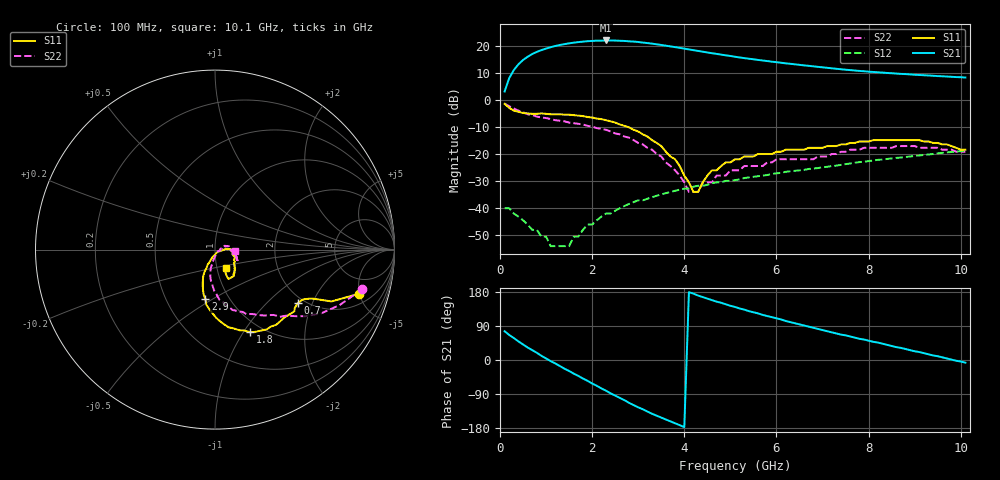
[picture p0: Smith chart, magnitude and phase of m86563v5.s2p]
!  MGA-86563 S PARAMETERS
!  Vd = 5 V  LAST UPDATED 12-19-94
# ghz s ma r 50
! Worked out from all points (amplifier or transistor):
!   101 points, 100 MHz to 10.1 GHz, reference 50 ohm
!   highest |S21| = 21.9 dB at 2.3 GHz (marker M1)
!   |S21| within 3 dB of that: 1 GHz to 3.993 GHz (2.992 GHz wide, 120 % of centre)
!   unconditionally stable (mu >= 1): start of sweep to end of sweep
!   at 1.7 GHz: K = 9.49, MAG = 23.1 dB, |S12| = -50.5 dB
!   at 5.1 GHz: K = 2.52, MAG = 15.9 dB, |S12| = -29.6 dB
!   at 10.1 GHz: K = 1.78, MAG = 8.3 dB, |S12| = -18.7 dB
!   lowest NFmin = 1.52 dB at 1.5 GHz
!   S11 on the Smith chart (normalised r, x): 100 MHz: 2.97, -4.96; 700 MHz: 1.84, -1.58; 1.8 GHz: 0.87, -1.07; 2.9 GHz: 0.78, -0.46; 10.1 GHz: 1.11, -0.23
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0.1  0.84 -17.0  1.42 76.0  0.01 15.0  0.85 -15.0
0.4  0.6 -27.0  4.5 49.0  0.007 -23.0  0.63 -36.0
0.7  0.55 -33.0  6.97 26.0  0.004 -20.0  0.52 -46.0
1  0.55 -41.0  8.77 4.0  0.003 -2.0  0.46 -53.0
1.3  0.54 -51.0  10.23 -16.0  0.002 37.0  0.41 -61.0
1.5  0.53 -57.0  10.97 -29.0  0.002 70.0  0.38 -66.0
1.8  0.5 -67.0  11.8 -49.0  0.004 91.0  0.35 -74.0
2.1  0.45 -77.0  12.28 -68.0  0.006 100.0  0.3 -81.0
2.3  0.42 -83.0  12.39 -81.0  0.008 102.0  0.28 -85.0
2.6  0.35 -93.0  12.23 -100.0  0.01 101.0  0.23 -91.0
2.9  0.28 -101.0  11.82 -119.0  0.013 101.0  0.18 -97.0
3.2  0.21 -109.0  11.09 -136.0  0.015 99.0  0.13 -101.0
3.5  0.14 -115.0  10.23 -152.0  0.018 97.0  0.09 -102.0
3.9  0.06 -112.0  9.05 -172.0  0.022 93.0  0.04 -91.0
4.3  0.02 -36.0  7.94 170.0  0.026 90.0  0.02 -23.0
4.7  0.05 1.0  7 154.0  0.03 86.0  0.04 11.0
5.1  0.08 2.0  6.21 140.0  0.033 81.0  0.05 20.0
5.8  0.1 -12.0  5.17 116.0  0.041 74.0  0.07 17.0
6.8  0.13 -33.0  4.13 85.0  0.054 62.0  0.08 0.0
7.4  0.15 -42.0  3.65 67.0  0.063 54.0  0.11 -10.0
8.5  0.18 -60.0  3.08 37.0  0.083 36.0  0.13 -24.0
10.1  0.12 -59.0  2.57 -7.0  0.116 5.0  0.11 -3.0
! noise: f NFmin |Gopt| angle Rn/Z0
0.1  3.78  0.66  -19  1.8
1.2  1.62  0.54  28  0.36
2.3  1.56  0.42  46  0.35
3.4  1.65  0.35  63  0.28
4.5  1.81  0.28  84  0.27
5.6  1.99  0.19  117  0.25
6.7  2.18  0.09  155  0.22
7.8  2.37  0.01  9  0.19
8.9  2.57  0.1  49  0.16
10.1  2.78  0.21  89  0.13
